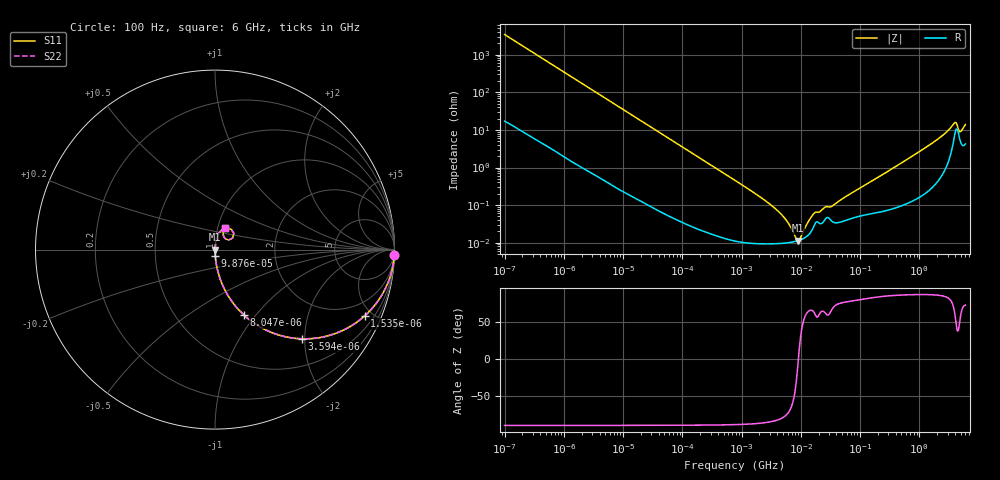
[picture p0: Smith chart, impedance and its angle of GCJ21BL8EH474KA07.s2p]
!Murata Part Number: GCJ21BL8EH474KA07
!These Parameters are Measured in Series Mode Connection
!Data Generated on Mar 13, 2026
!  o--ll--o
!Port1  Port2
!  o------o
!Operation Temp=25[degC], DC Bias Voltage=0[V]
!Freq. Start=100[Hz] Stop=6[GHz] 401[Steps]
# Hz S RI R 50
!Freq.(Hz) S11(Real) S11(Imag) S21(Real) S21(Imag) S12(Real) S12(Imag) S22(Real) S22(Imag)
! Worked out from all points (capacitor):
!   401 points, 100 Hz to 6 GHz, reference 50 ohm
!   read as one part in series: C = 463 nF near 109 Hz
!   lowest |Z| = 11.5 mohm at 9.09 MHz (marker M1)
!   series resonance near 9.106 MHz, so ESL is about 660 pH
!   S11 on the Smith chart (normalised r, x): 100 Hz: 1, -69; 1.535 kHz: 1.03, -4.51; 3.594 kHz: 1.01, -1.93; 8.047 kHz: 1.01, -0.87; 98.76 kHz: 1.00, -0.07; 6 GHz: 1.08, +0.26
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100  0.999 -0.0291  0.000993 0.0291  0.000993 0.0291  0.999 -0.0291
458  0.982 -0.1304  0.018 0.1304  0.018 0.1304  0.982 -0.1304
1535  0.8344 -0.3689  0.1656 0.3689  0.1656 0.3689  0.8344 -0.3689
2008  0.7475 -0.4315  0.2525 0.4315  0.2525 0.4315  0.7475 -0.4315
3594  0.4832 -0.4967  0.5168 0.4967  0.5168 0.4967  0.4832 -0.4967
8047  0.1596 -0.363  0.8404 0.363  0.8404 0.363  0.1596 -0.363
15062  0.0524 -0.2195  0.9476 0.2195  0.9476 0.2195  0.0524 -0.2195
40335  0.00819 -0.0862  0.9918 0.0862  0.9918 0.0862  0.00819 -0.0862
98762  0.00162 -0.0356  0.9984 0.0356  0.9984 0.0356  0.00162 -0.0356
774597  0.000132 -0.00456  0.9999 0.00456  0.9999 0.00456  0.000132 -0.00456
4060267  9.52e-05 -0.000706  0.9999 0.000706  0.9999 0.000706  9.52e-05 -0.000706
5809218  9.95e-05 -0.000367  0.9999 0.000367  0.9999 0.000367  9.95e-05 -0.000367
8311524  0.00011 -7.28e-05  0.9999 7.28e-05  0.9999 7.28e-05  0.00011 -7.28e-05
9090158  0.000115 -1.4e-06  0.9999 1.4e-06  0.9999 1.4e-06  0.000115 -1.4e-06
1.555665e7  0.00022 0.000476  0.9998 -0.000476  0.9998 -0.000476  0.00022 0.000476
2.545746e7  0.000409 0.000779  0.9996 -0.000779  0.9996 -0.000779  0.000409 0.000779
3.482834e7  0.000358 0.000905  0.9996 -0.000905  0.9996 -0.000905  0.000358 0.000905
3.124326e8  0.00082 0.00831  0.9992 -0.00831  0.9992 -0.00831  0.00082 0.00831
1.791126e9  0.00564 0.0481  0.9944 -0.0481  0.9944 -0.0481  0.00564 0.0481
3.8344e9  0.0685 0.1202  0.9315 -0.1202  0.9315 -0.1202  0.0685 0.1202
5.016141e9  0.0491 0.0708  0.9509 -0.0708  0.9509 -0.0708  0.0491 0.0708
6e9  0.0558 0.1197  0.9442 -0.1197  0.9442 -0.1197  0.0558 0.1197
